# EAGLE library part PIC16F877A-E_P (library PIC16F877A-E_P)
8-bit Microcontrollers - MCU 14KB 368 RAM 33 I/O Source: Datasheet
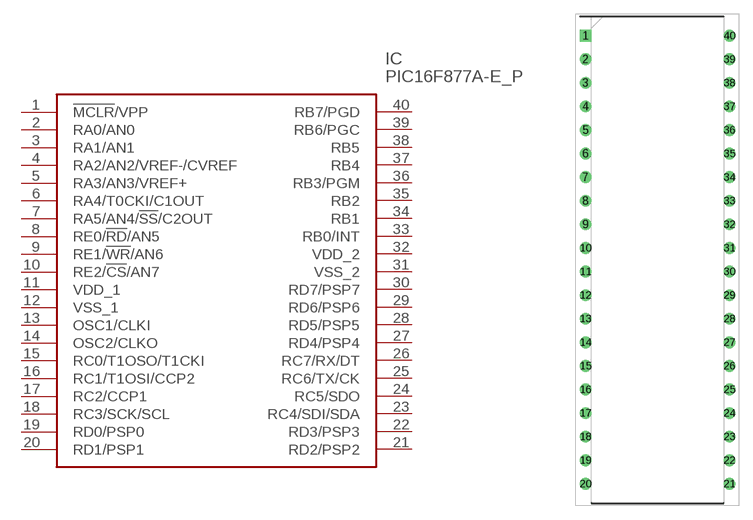
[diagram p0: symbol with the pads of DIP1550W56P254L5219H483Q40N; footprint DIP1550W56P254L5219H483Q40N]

Designator prefix IC

## PIC16F877A-E_P (Description: 8-bit Microcontrollers - MCU 14KB 368 RAM 33 I/O; Height: 4.83mm; Manufacturer_Name: Microchip; Manufacturer_Part_Number: PIC16F877A-E/P; Mouser_Part_Number: 579-PIC16F877A-E/P; Mouser_Price-Stock: https://www.mouser.co.uk/ProductDetail/Microchip-Technology/PIC16F877A-E-P?qs=oKK8NaWdAJsQw%252B2Y417CHw%3D%3D)  [DIP1550W56P254L5219H483Q40N]
1  !MCLR!/VPP
2  RA0/AN0
3  RA1/AN1
4  RA2/AN2/VREF-/CVREF
5  RA3/AN3/VREF+
6  RA4/T0CKI/C1OUT
7  RA5/AN4/!SS!/C2OUT
8  RE0/!RD!/AN5
9  RE1/!WR!/AN6
10  RE2/!CS!/AN7
11  VDD_1
12  VSS_1
13  OSC1/CLKI
14  OSC2/CLKO
15  RC0/T1OSO/T1CKI
16  RC1/T1OSI/CCP2
17  RC2/CCP1
18  RC3/SCK/SCL
19  RD0/PSP0
20  RD1/PSP1
21  RD2/PSP2
22  RD3/PSP3
23  RC4/SDI/SDA
24  RC5/SDO
25  RC6/TX/CK
26  RC7/RX/DT
27  RD4/PSP4
28  RD5/PSP5
29  RD6/PSP6
30  RD7/PSP7
31  VSS_2
32  VDD_2
33  RB0/INT
34  RB1
35  RB2
36  RB3/PGM
37  RB4
38  RB5
39  RB6/PGC
40  RB7/PGD

## Footprint DIP1550W56P254L5219H483Q40N (pad centres in mm)
40-Lead Plastic Dual In-line (P) &ndash; 600 mil (PDIP)
drill 0.76 pad 1.16 square: 1 -7.748,24.13
drill 0.76 pad 1.16: 2 -7.748,21.59; 3 -7.748,19.05; 4 -7.748,16.51; 5 -7.748,13.97; 6 -7.748,11.43; 7 -7.748,8.89; 8 -7.748,6.35; 9 -7.748,3.81; 10 -7.748,1.27; 11 -7.748,-1.27; 12 -7.748,-3.81; 13 -7.748,-6.35; 14 -7.748,-8.89; 15 -7.748,-11.43; 16 -7.748,-13.97; 17 -7.748,-16.51; 18 -7.748,-19.05; 19 -7.748,-21.59; 20 -7.748,-24.13; 21 7.748,-24.13; 22 7.748,-21.59; 23 7.748,-19.05; 24 7.748,-16.51; 25 7.748,-13.97; 26 7.748,-11.43; 27 7.748,-8.89; 28 7.748,-6.35; 29 7.748,-3.81; 30 7.748,-1.27; 31 7.748,1.27; 32 7.748,3.81; 33 7.748,6.35; 34 7.748,8.89; 35 7.748,11.43; 36 7.748,13.97; 37 7.748,16.51; 38 7.748,19.05; 39 7.748,21.59; 40 7.748,24.13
